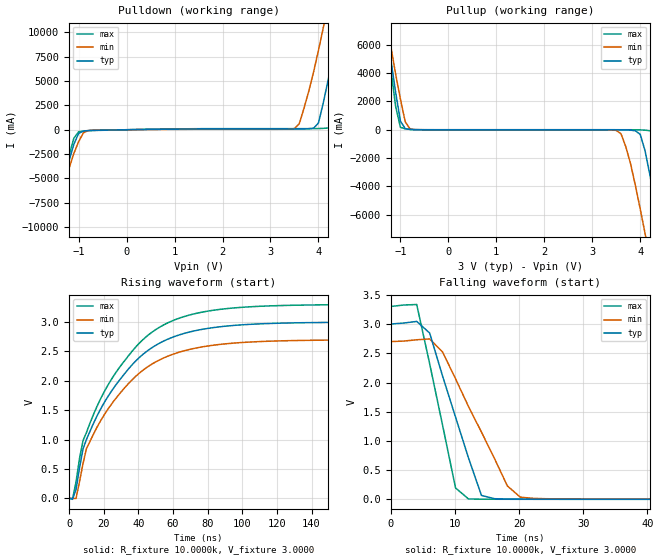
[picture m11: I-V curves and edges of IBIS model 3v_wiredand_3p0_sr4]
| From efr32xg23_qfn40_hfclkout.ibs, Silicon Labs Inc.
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|   Model 3v_wiredand_3p0_sr4
[Model]  3v_wiredand_3p0_sr4
Model_type Output
Polarity   Inverting
Enable   Active-Low
C_comp   1.6300pF   1.4000pF   2.7000pF
[Temperature Range]   25.0000   0.1250k   -40.0000
[Pullup Reference]   3.0000V   2.7000V   3.3000V
[Pulldown Reference]   0.0V   0.0V   0.0V
[POWER Clamp Reference]   3.0000V   2.7000V   3.3000V
[GND Clamp Reference]   0.0V   0.0V   0.0V
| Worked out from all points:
|   slope of the pulldown table from 0 to 0.45 V, typ, clamps not added: 13.2 ohm
|   rising waveform, R_fixture 10.0000k, V_fixture 3.0000: 20-80 % time 34.1ns typ, 34ns min, 34.5ns max; typ from 0.003 V to 3 V
|   falling waveform, R_fixture 10.0000k, V_fixture 3.0000: 20-80 % time 5.18ns typ, 7.17ns min, 3.8ns max; typ from 3 V to 0.003 V
[Pulldown]
|Voltage   I(typ)   I(min)   I(max)
-3V       -32.58A    -30.59A    -34.31A
-1.6V     -10.64A    -10.81A    -10.62A
-1V       -369.5mA   -1.223A    -213mA
-700mV    -60.92mA   -44.3mA    -77.77mA
3.5V      79.82mA    115.9mA    114.1mA
3.7V      85.6mA     2.224A     114.4mA
4V        694.1mA    8.145A     121.6mA
4.1V      2.74A      10.47A     138.5mA
4.3V      7.585A     15.22A     289.6mA
4.4V      10.25A     17.53A     1.779A
4.7V      18.35A     24.09A     10.24A
6V        48.97A     49.46A     46.24A
[Pullup]
|Voltage   I(typ)   I(min)   I(max)
-3V       48.87A     43.59A     53.88A
-1.3V     7.504A     8.096A     7.139A
-1V       614.1mA    2.175A     173.1mA
-700mV    6.154mA    10.05mA    6.499mA
3.5V      -715.9uA   -46.84mA   -9.332nA
3.7V      -7.458mA   -1.208A    -41.68uA
4V        -326.2mA   -5.611A    -8.238mA
4.1V      -1.482A    -7.329A    -28.72mA
4.3V      -4.973A    -10.8A     -136.7mA
4.4V      -6.846A    -12.49A    -837.1mA
4.8V      -14.25A    -18.59A    -8.585A
6V        -32.58A    -34.37A    -29.65A
[Ramp]
| variable   typ   min   max
dV/dt_r  5.8727u/18.9868n   52.6514u/20.8980n   8.1487u/19.3180n
dV/dt_f  1.7980/5.1770n   1.6171/7.1748n   1.9783/3.8005n
R_load = 10.0000k
[Rising Waveform]
R_fixture= 10.0000k
V_fixture= 3.0000
V_fixture_min= 2.7000
V_fixture_max= 3.3000
|time   V(typ)   V(min)   V(max)
0s        3.402mV    4.707mV    2.76mV
2.02ns    -9.43mV    666.2uV    -15.16mV
4.04ns    150.7mV    -593.9uV   279.9mV
8.081ns   843.5mV    593.6mV    984.2mV
10.1ns    1.006V     854mV      1.125V
20.2ns    1.625V     1.417V     1.808V
38.38ns   2.335V     2.075V     2.572V
52.53ns   2.646V     2.361V     2.917V
94.95ns   2.942V     2.642V     3.24V
200ns     2.999V     2.699V     3.299V
[Falling Waveform]
R_fixture= 10.0000k
V_fixture= 3.0000
V_fixture_min= 2.7000
V_fixture_max= 3.3000
|time   V(typ)   V(min)   V(max)
0s        3V         2.7V       3.3V
4.04ns    3.044V     2.731V     3.333V
6.061ns   2.845V     2.744V     2.32V
8.081ns   2.108V     2.52V      1.267V
10.1ns    1.407V     2.063V     197mV
12.12ns   708.8mV    1.589V     9.143mV
14.14ns   69.5mV     1.152V     5.4mV
18.18ns   8.189mV    231.7mV    3.834mV
22.22ns   5.508mV    18.93mV    3.363mV
200ns     3.404mV    4.71mV     2.761mV
